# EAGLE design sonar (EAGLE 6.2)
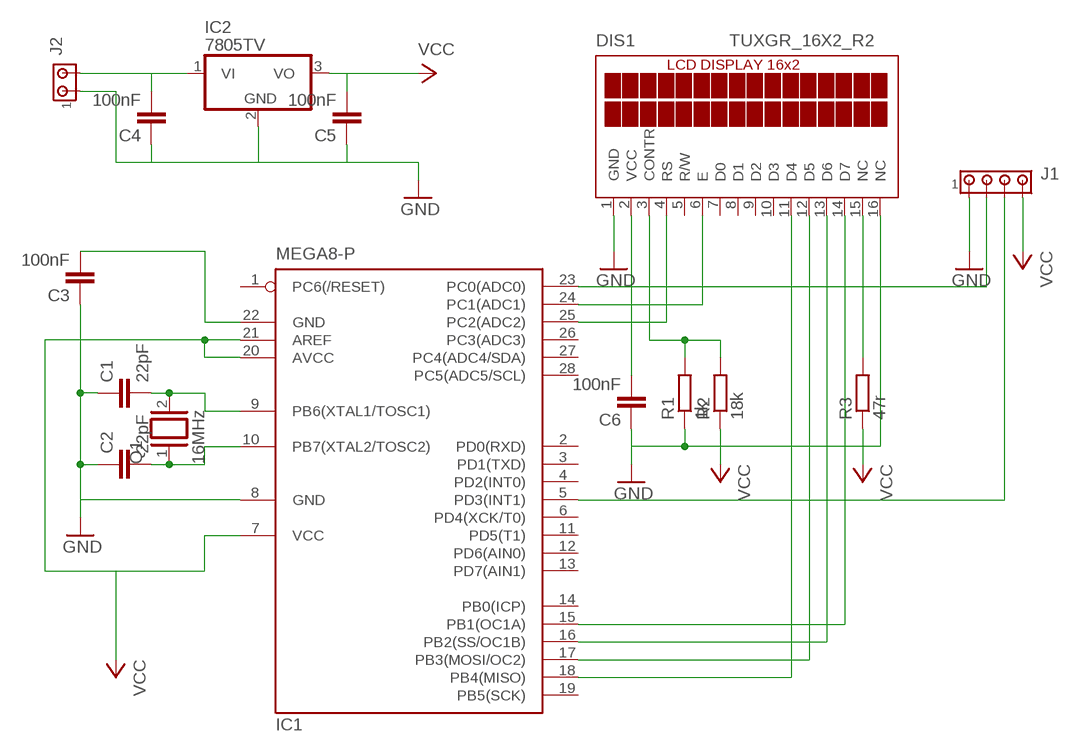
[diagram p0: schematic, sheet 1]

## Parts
C1  22pF  C2.5/2  [C2.5-2]
C2  22pF  C2.5/2  [C2.5-2]
C3  100nF  C5/2.5  [C5B2.5]
C4  100nF  C5/2.5  [C5B2.5]
C5  100nF  C5/2.5  [C5B2.5]
C6  100nF  C2.5/2  [C2.5-2]
DIS1  TUXGR_16X2_R2  [TUXGR_16X2_R2]
IC1  MEGA8-P  [DIL28-3]
IC2  7805TV  [TO220V]
J1  MTA04-100  [10X04MTA]
J2  MTA02-156  [1X2MTA]
Q1  16MHz  XTAL/S  [QS]
R1  1k  R-EU_0204/7  [0204/7]
R2  18k  R-EU_0204/7  [0204/7]
R3  47r  R-EU_0204/7  [0204/7]

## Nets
GND: C1.1 C2.1 C3.1 C4.1 C5.1 C6.1 DIS1.1(GND) DIS1.16(NC) IC1.8(GND) IC2.2(GND) J1.1 J2.1 R1.1
N$1: DIS1.11(D4) IC1.18(PB4(MISO))
N$2: DIS1.12(D5) IC1.17(PB3(MOSI/OC2))
N$3: DIS1.13(D6) IC1.16(PB2(SS/OC1B))
N$4: DIS1.14(D7) IC1.15(PB1(OC1A))
N$5: DIS1.4(RS) IC1.25(PC2(ADC2))
N$6: DIS1.6(E) IC1.24(PC1(ADC1))
N$7: C1.2 IC1.9(PB6(XTAL1/TOSC1)) Q1.2
N$8: C2.2 IC1.10(PB7(XTAL2/TOSC2)) Q1.1
N$9: C4.2 IC2.1(VI) J2.2
N$10: C3.2 IC1.22(GND)
N$11: IC1.23(PC0(ADC0)) J1.2
N$12: IC1.5(PD3(INT1)) J1.3
N$14: C6.2 DIS1.2(VCC)
N$15: DIS1.3(CONTR) R1.2 R2.2
N$16: DIS1.15(NC) R3.2
VCC: C5.2 IC1.7(VCC) IC1.20(AVCC) IC1.21(AREF) IC2.3(VO) J1.4 R2.1 R3.1
Unconnected: DIS1.5(R/W) DIS1.7(D0) DIS1.8(D1) DIS1.9(D2) DIS1.10(D3) IC1.1(PC6(/RESET)) IC1.2(PD0(RXD)) IC1.3(PD1(TXD)) IC1.4(PD2(INT0)) IC1.6(PD4(XCK/T0)) IC1.11(PD5(T1)) IC1.12(PD6(AIN0)) IC1.13(PD7(AIN1)) IC1.14(PB0(ICP)) IC1.19(PB5(SCK)) IC1.26(PC3(ADC3)) IC1.27(PC4(ADC4/SDA)) IC1.28(PC5(ADC5/SCL))

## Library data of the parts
C1-C6 = capacitor-wima:C: CAPACITOR
DIS1 = display-lcd:TUXGR_16X2_R2: Tuxgraphics LCD display 16x2 characters reflective, without background light Source: tuxgr_12x2_r2.pdf; OC_FARNELL: unknown; OC_NEWARK: unknown
IC1 = atmel:MEGA8-P: MICROCONTROLLER 8 Kbytes FLASH, 1 kbytes SRAM, 512 bytes EEPROM, USART, 4-channel 10 bit ADC, 2-channel 8 bit ADC Pin compatible with Atmega48, ATMega88, ATMega168 Source: avr.lbr; OC_FARNELL: unknown; OC_NEWARK: unknown
IC2 = linear:78*: Positive VOLTAGE REGULATOR Source: http://cache.national.com/ds/LM/LM78L05.pdf http://www.fairchildsemi.com/ds/LM/LM7805.pdf
J1 = con-amp:MTA04-100: AMP connector
J2 = con-amp:MTA02-156: AMP connector
Q1 = special:XTAL/S: CRYSTAL
R1-R3 = rcl:R-EU_: RESISTOR, European symbol

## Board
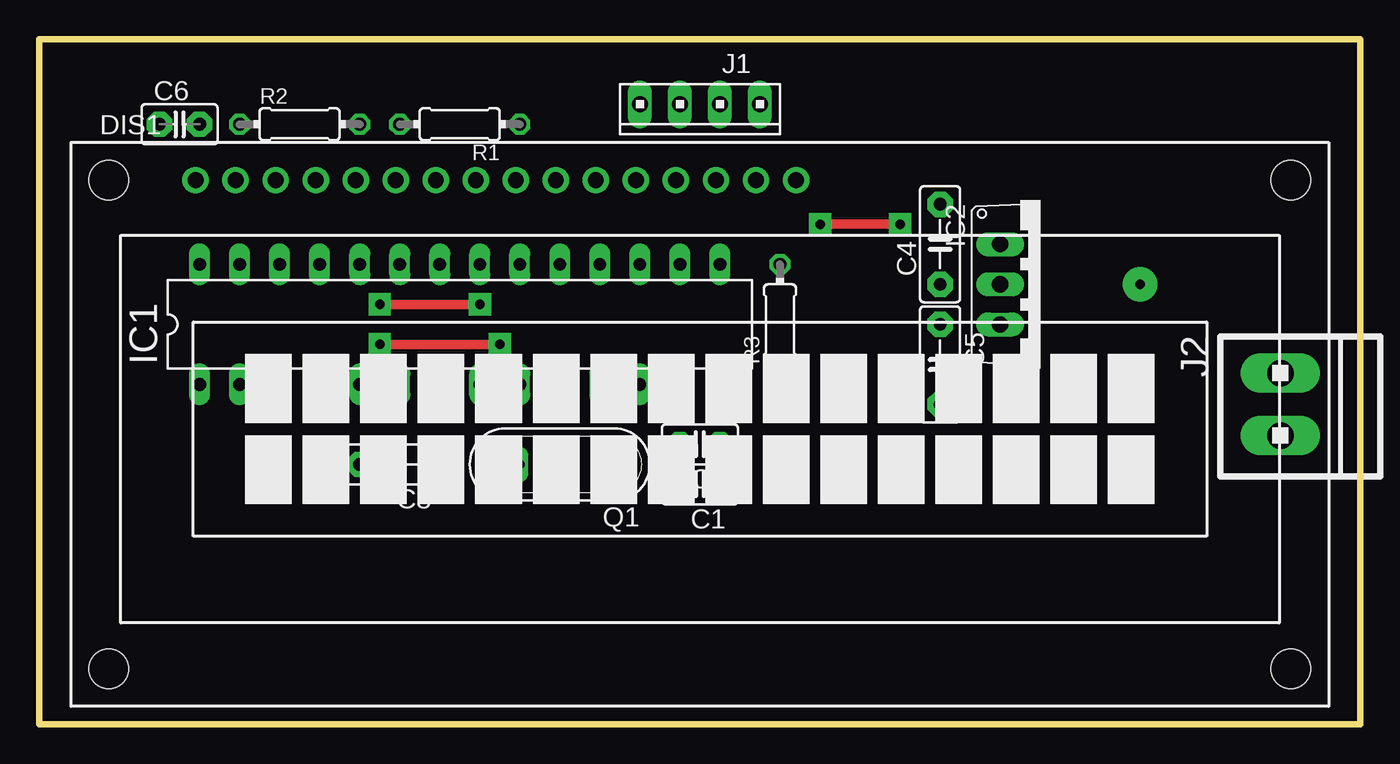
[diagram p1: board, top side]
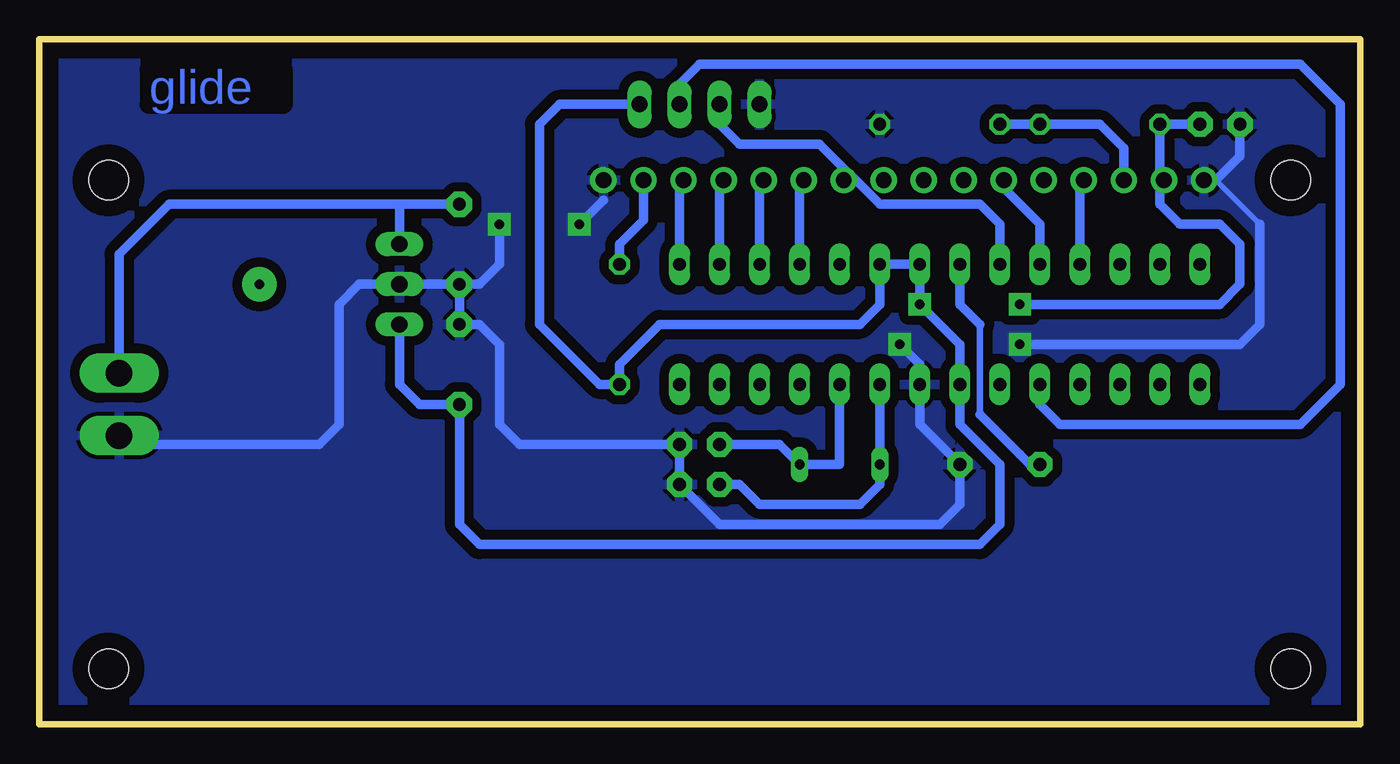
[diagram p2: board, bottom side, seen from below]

Size 83.8 x 43.48 mm. Coordinates in mm from the lower left corner, seen from the top.
Outline: 0,0 83.8,0 83.8,43.48 0,43.48 0,0
Copper layers (1*16): Top 0.035mm / dielectric 1.5mm / Bottom 0.035mm
Design rules: minimum track width 10mil, minimum drill 24mil, track to track 8mil, track to pad 8mil, pad to pad 8mil, via to via 8mil, smd to smd 8mil, copper to edge 40mil, drill to drill 8mil, minimum pad ring 10mil, minimum via ring 16mil, stop-mask expansion 4mil, vias tented up to drill 0mil, thermal gap 10mil

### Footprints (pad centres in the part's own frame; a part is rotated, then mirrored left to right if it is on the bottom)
C2.5-2 = drill 0.813 pad 1.6 octagon: 1 -1.27,0; 2 1.27,0
C5B2.5 = drill 0.813 pad 1.6 octagon: 1 -2.54,0; 2 2.54,0
TUXGR_16X2_R2 = drill 1 pad 1.676: 1 -32,15.5; 2 -29.46,15.5; 3 -26.92,15.5; 4 -24.38,15.5; 5 -21.84,15.5; 6 -19.3,15.5; 7 -16.76,15.5; 8 -14.22,15.5; 9 -11.68,15.5; 10 -9.14,15.5; 11 -6.6,15.5; 12 -4.06,15.5; 13 -1.52,15.5; 14 1.02,15.5; 15 3.56,15.5; 16 6.1,15.5 | hole 2.5: -37.5,-15.5; 37.5,-15.5; -37.5,15.5; 37.5,15.5
DIL28-3 = drill 0.813 long: 1 -16.51,-3.81; 2 -13.97,-3.81; 3 -11.43,-3.81; 4 -8.89,-3.81; 5 -6.35,-3.81; 6 -3.81,-3.81; 7 -1.27,-3.81; 8 1.27,-3.81; 9 3.81,-3.81; 10 6.35,-3.81; 11 8.89,-3.81; 12 11.43,-3.81; 13 13.97,-3.81; 14 16.51,-3.81; 15 16.51,3.81; 16 13.97,3.81; 17 11.43,3.81; 18 8.89,3.81; 19 6.35,3.81; 20 3.81,3.81; 21 1.27,3.81; 22 -1.27,3.81; 23 -3.81,3.81; 24 -6.35,3.81; 25 -8.89,3.81; 26 -11.43,3.81; 27 -13.97,3.81; 28 -16.51,3.81
TO220V = drill 1.016 long: 1 -2.54,-2.54; 2 0,-2.54; 3 2.54,-2.54
10X04MTA = drill 1.016 long: 1 3.81,0; 2 1.27,0; 3 -1.27,0; 4 -3.81,0
1X2MTA = drill 1.676 long: 1 1.981,0; 2 -1.981,0
QS = drill 0.61 long: 1 -2.54,0; 2 2.54,0
0204/7 = drill 0.813 octagon: 1 -3.81,0; 2 3.81,0

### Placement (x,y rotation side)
C1  41.91,15.24 180 top
C2  41.91,17.78 180 top
C3  22.86,16.51 180 top
C4  57.15,30.48 90 top
C5  57.15,22.86 270 top
C6  8.89,38.1 0 top
DIS1  41.91,19.05 0 top
IC1  26.67,25.4 0 top
IC2  63.5,27.94 270 top
J1  41.91,39.37 180 top
J2  78.74,20.32 270 top
Q1  33.02,16.51 180 top
R1  26.67,38.1 180 top
R2  16.51,38.1 0 top
R3  46.99,25.4 90 top

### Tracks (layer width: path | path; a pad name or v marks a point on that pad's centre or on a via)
GND  (via drill 0.6, 0.6 pad 1.42)
  Top 0.61: v21.59,24.13 v29.21,24.13 | v49.53,31.75 v54.61,31.75
  Bottom 0.305: 9.15,34.55 6.35,31.75
  Bottom 0.61: 80.72,18.34 J2.1 78.18,17.78 66.04,17.78 64.77,19.05 64.77,26.67 63.5,27.94 IC2.2 C4.1 | C4.1 C5.1 55.88,25.4 54.61,24.13 54.61,19.05 53.34,17.78 C2.1 C1.1 40.64,12.7 26.67,12.7 25.4,13.97 C3.1 27.94,19.05 IC1.8 27.94,22.86 v29.21,24.13 | DIS1.1 9.15,34.55 7.62,36.08 C6.1 | 6.35,31.75 6.35,25.4 7.62,24.13 v21.59,24.13 | 48.01,33.27 v49.53,31.75 | v54.61,31.75 54.61,29.21 55.88,27.94 C4.1
  pour Bottom (isolate 0.61): 0,43.18 83.82,43.18 83.82,0 0,0
N$1
  Bottom 0.61: IC1.18 35.56,34.3 DIS1.11
N$2
  Bottom 0.61: IC1.17 38.1,34.3 DIS1.12
N$3
  Bottom 0.61: IC1.16 40.64,34.3 DIS1.13
N$4
  Bottom 0.61: IC1.15 43.18,34.3 DIS1.14
N$5
  Bottom 0.61: IC1.25 17.78,34.3 DIS1.4
N$6
  Bottom 0.61: IC1.24 20.32,31.75 22.86,34.3 DIS1.6
N$7
  Bottom 0.61: IC1.9 Q1.2 30.48,15.24 31.75,13.97 38.1,13.97 39.37,15.24 C1.2
N$8
  Bottom 0.61: IC1.10 33.02,16.51 Q1.1 36.83,17.78 C2.2
N$9
  Bottom 0.61: C4.2 60.96,33.02 | 60.96,33.02 75.56,33.02 78.74,29.84 J2.2 | IC2.1 60.96,33.02
N$10
  Bottom 0.406: 24.13,19.68 24.13,25.4
  Bottom 0.61: C3.2 20.95,16.51 21.59,17.14 24.13,19.68 | 24.13,25.4 25.4,26.67 IC1.22
N$11
  Bottom 0.61: IC1.23 22.86,31.75 24.13,33.02 30.48,33.02 34.29,36.83 39.37,36.83 40.64,38.1 J1.2
N$12
  Bottom 0.61: IC1.5 20.32,20.32 19.05,19.05 3.81,19.05 1.27,21.59 1.27,39.37 3.81,41.91 41.91,41.91 43.18,40.64 J1.3
N$13  (via drill 0.6 pad 2.18)
  other vias: 69.85,27.94
N$14
  Bottom 0.61: C6.2 12.7,38.1 12.7,34.8 DIS1.2
N$15
  Bottom 0.61: DIS1.3 14.99,36.58 16.51,38.1 R1.2 R2.2
N$16
  Bottom 0.61: DIS1.15 45.47,32 46.99,30.48 R3.2
VCC  (via drill 0.6)
  Top 0.61: v27.94,26.67 v21.59,26.67
  Bottom 0.61: IC2.3 60.96,21.59 59.69,20.32 C5.2 57.15,12.7 55.88,11.43 24.13,11.43 22.86,12.7 22.86,16.51 25.4,19.05 IC1.7 25.4,24.13 v27.94,26.67 IC1.21 IC1.20 30.48,26.67 31.75,25.4 44.45,25.4 46.99,22.86 R3.1 48.26,21.59 52.07,25.4 52.07,38.1 50.8,39.37 J1.4 | v21.59,26.67 8.89,26.67 7.62,27.94 7.62,30.48 8.89,31.75 11.43,31.75 12.7,33.02 R2.1

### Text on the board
Bottom: glide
